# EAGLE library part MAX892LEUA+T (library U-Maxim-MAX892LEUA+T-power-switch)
MAX891L / MAX892L Current-Limited, High-Side P-Channel Switch with Thermal Shutdown
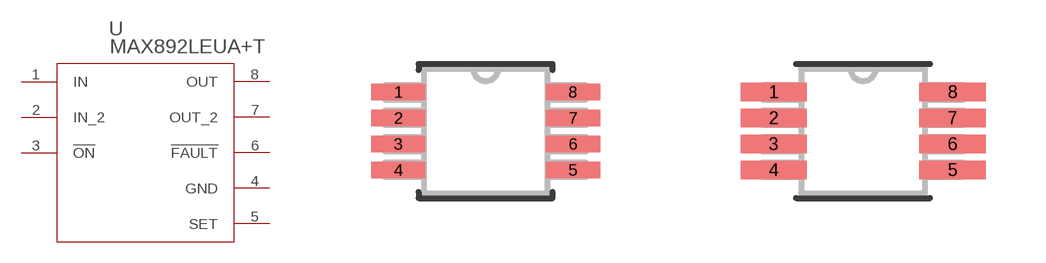
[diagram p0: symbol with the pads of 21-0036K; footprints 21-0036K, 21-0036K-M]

Designator prefix U

## MAX892LEUA+T (MANUFACTURER_PART_NUMBER: MAX892LEUA+T; VENDOR: Maxim Integrated Products)  [21-0036K]
1  IN  pwr
2  IN_2  pwr
3  !ON  in
4  GND  pwr
5  SET  in
6  !FAULT  out
7  OUT_2  pwr
8  OUT  pwr

## MAX892LEUA+T21-0036K-M (MANUFACTURER_PART_NUMBER: MAX892LEUA+T; VENDOR: Maxim Integrated Products)  [21-0036K-M]
1  IN_2  pwr
2  IN  pwr
3  !ON  in
4  GND  pwr
5  SET  in
6  !FAULT  out
7  OUT_2  pwr
8  OUT  pwr

## MAX892LEUA+T21-0036K-L (MANUFACTURER_PART_NUMBER: MAX892LEUA+T; VENDOR: Maxim Integrated Products)  [21-0036K-L]
Pads as for 21-0036K-M

## Footprint 21-0036K (pad centres in mm)
smd 1.36 x 0.416: 1 -2.184,0.975; 2 -2.184,0.325; 3 -2.184,-0.325; 4 -2.184,-0.975; 5 2.184,-0.975; 6 2.184,-0.325; 7 2.184,0.325; 8 2.184,0.975

## Footprint 21-0036K-M (pad centres in mm)
smd 1.66 x 0.456: 1 -2.234,0.975; 2 -2.234,0.325; 3 -2.234,-0.325; 4 -2.234,-0.975; 5 2.234,-0.975; 6 2.234,-0.325; 7 2.234,0.325; 8 2.234,0.975

## Footprint 21-0036K-L (pad centres in mm)
smd 1.06 x 0.376: 1 -2.134,0.975; 2 -2.134,0.325; 3 -2.134,-0.325; 4 -2.134,-0.975; 5 2.134,-0.975; 6 2.134,-0.325; 7 2.134,0.325; 8 2.134,0.975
